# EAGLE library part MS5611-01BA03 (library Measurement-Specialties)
Variometer Module, with stainless steel cap
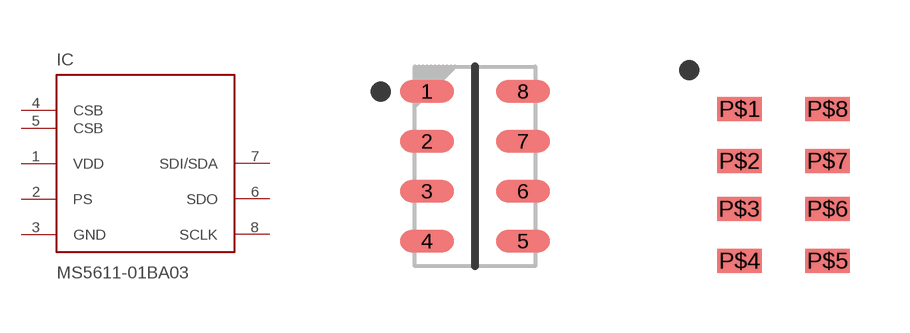
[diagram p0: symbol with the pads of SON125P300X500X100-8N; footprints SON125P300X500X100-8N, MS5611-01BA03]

Designator prefix IC

## MS5611-01BA03UNO  [SON125P300X500X100-8N]
1  VDD  pwr
2  PS  in
3  GND  pwr
4  CSB  in
5  CSB  in
6  SDO  out
7  SDI/SDA
8  SCLK  in

## MS5611-01BA03  [MS5611-01BA03]
P$1  VDD  pwr
P$2  PS  in
P$3  GND  pwr
P$4  CSB  in
P$5  CSB  in
P$6  SDO  out
P$7  SDI/SDA
P$8  SCLK  in

## Footprint SON125P300X500X100-8N (pad centres in mm)
SON,1.25mm,pitch;8 pin,3.00mm W X 5.00mm L X 1.00mm H body
smd 1.35 x 0.55: 1 -1.2,1.875; 2 -1.2,0.625; 3 -1.2,-0.625; 4 -1.2,-1.875; 5 1.2,-1.875; 6 1.2,-0.625; 7 1.2,0.625; 8 1.2,1.875

## Footprint MS5611-01BA03 (pad centres in mm)
SON,1.25mm,pitch;8 pin,3.00mm W X 5.00mm L X 1.00mm H body
smd 1.1 x 0.6: P$1 -1.1,1.9; P$2 -1.1,0.6; P$3 -1.11,-0.6; P$4 -1.1,-1.9; P$5 1.1,-1.9; P$6 1.1,-0.6; P$7 1.1,0.6; P$8 1.1,1.9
